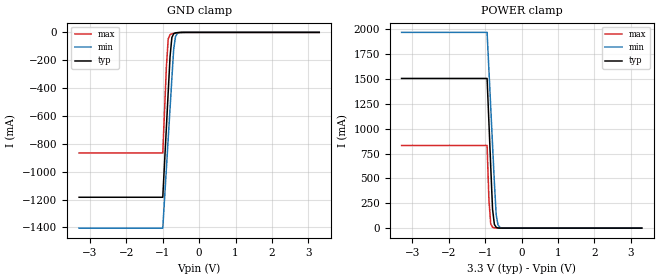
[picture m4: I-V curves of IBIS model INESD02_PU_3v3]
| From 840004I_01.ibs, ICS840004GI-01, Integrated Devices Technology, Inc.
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[Model] INESD02_PU_3v3
Model_type   Input
Polarity   Non-Inverting
Vinl = 0.80V
Vinh = 2.0V
|   typ   min   max
C_comp   2pF   1.5pF   2.5pF
|   typ   min   max
[Voltage range]  3.3V   3.15V   3.45V
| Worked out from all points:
|   GND clamp passes 1 mA (typ) near -0.56 V on its own axis
|   POWER clamp passes 1 mA (typ) near -0.61 V on its own axis
[GND_clamp]
|Voltage   I(typ)   I(min)   I(max)
-3.3V     -1.184A    -1.405A    -865.6mA
-1V       -1.184A    -1.405A    -865.6mA
-900mV    -678.5mA   -975.1mA   -244.1mA
-850mV    -426.2mA   -760.2mA   -46.92mA
-800mV    -174mA     -545.4mA   -16.17mA
-750mV    -37.03mA   -330.8mA   -9.981mA
-700mV    -9.767mA   -120.3mA   -7.122mA
-650mV    -3.616mA   -29.78mA   -4.922mA
-600mV    -1.7mA     -7.594mA   -3.115mA
-400mV    -123.9uA   -126uA     -173.9uA
3.3V      1.866nA    3.949uA    0A
[POWER_clamp]
|Voltage   I(typ)   I(min)   I(max)
-3.3V     1.506A     1.97A      832.1mA
-950mV    1.506A     1.97A      832.1mA
-900mV    1.063A     1.592A     287.2mA
-850mV    620.4mA    1.215A     41.77mA
-800mV    191.5mA    837.4mA    8.692mA
-750mV    37.69mA    460.1mA    3.262mA
-700mV    8.032mA    133.8mA    1.662mA
-650mV    2.005mA    32.58mA    840.1uA
-600mV    607uA      8.009mA    378.6uA
-450mV    33.11uA    139.8uA    23.88uA
3.3V      -71.13uA   -77.46uA   -62.11uA
